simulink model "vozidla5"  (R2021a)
settings: Solver=VariableStepAuto  StartTime=0.0  StopTime=10.0  RelTol=1e-3
undefined symbols (not defined in the file or in its folder): ABK5, BC5, CC5, conds05, conds5, DC5
libraries: simulink x1

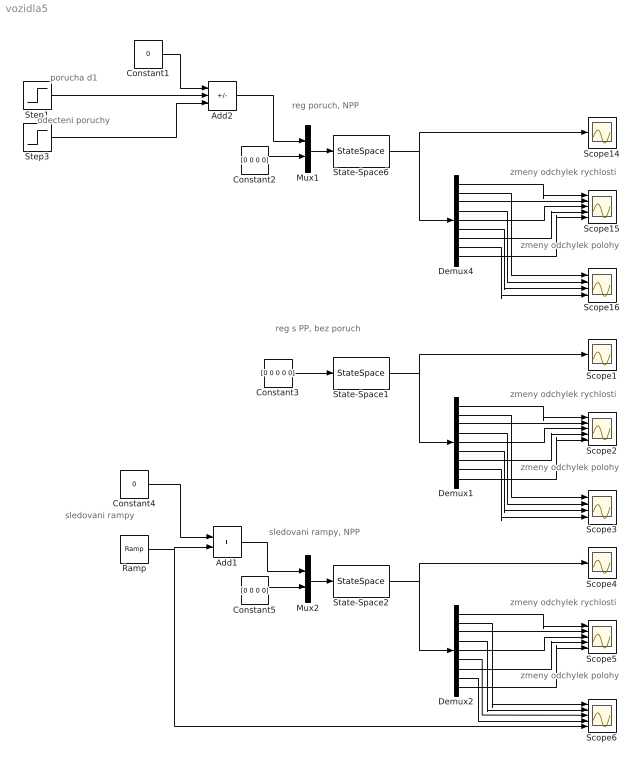
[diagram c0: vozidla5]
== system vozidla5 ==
  note: sledovani rampy
  note: reg poruch, NPP
  note: reg s PP, bez poruch
  note: odecteni poruchy
  note: porucha d1
  note: zmeny odchylek rychlosti
  note: zmeny odchylek polohy
  note: zmeny odchylek polohy
  note: zmeny odchylek rychlosti
  note: zmeny odchylek polohy
  note: sledovani rampy, NPP
  note: zmeny odchylek rychlosti
  Add1 : Sum
  Add2 : Sum  Inputs=++-
  Constant1 : Constant  Value=0
  Constant2 : Constant  Value=[0 0 0 0]
  Constant3 : Constant  Value=[0 0 0 0 0]
  Constant4 : Constant  Value=0
  Constant5 : Constant  Value=[0 0 0 0]
  Demux1 : Demux  Outputs=9
  Demux2 : Demux  Outputs=9
  Demux4 : Demux  Outputs=9
  Mux1 : Mux  Inputs=2
  Mux2 : Mux  Inputs=2
  Ramp : simulink/Sources/Ramp  slope=1  start=0  InitialOutput=0
  Scope1 : Scope
  Scope14 : Scope
  Scope{2,5..6,15} (4 alike) : Scope  NumInputPorts=5
  Scope16 : Scope  NumInputPorts=4
  Scope3 : Scope  NumInputPorts=4
  Scope4 : Scope
  State-Space1 : StateSpace  A=ABK5  B=BC5  C=CC5  D=DC5  InitialCondition=conds5
  State-Space2 : StateSpace  A=ABK5  B=BC5  C=CC5  D=DC5  InitialCondition=conds05
  State-Space6 : StateSpace  A=ABK5  B=BC5  C=CC5  D=DC5  InitialCondition=conds05
  Step1 : Step  Time=5  After=2  SampleTime=0
  Step3 : Step  Time=6  After=2  SampleTime=0
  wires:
  Demux4/5 -> Scope15/3
  Demux4/1 -> Scope15/1
  State-Space6/1 -> Demux4/1, Scope14/1
  Step1/1 -> Add2/2
  Add2/1 -> Mux1/1
  Mux1/1 -> State-Space6/1
  Step3/1 -> Add2/3
  Demux4/3 -> Scope15/2
  Constant1/1 -> Add2/1
  Constant2/1 -> Mux1/2
  Demux4/7 -> Scope15/4
  Demux4/9 -> Scope15/5
  Demux4/2 -> Scope16/1
  Demux4/4 -> Scope16/2
  Demux4/6 -> Scope16/3
  Demux4/8 -> Scope16/4
  Demux1/6 -> Scope3/3
  Demux1/4 -> Scope3/2
  Demux1/7 -> Scope2/4
  Demux1/8 -> Scope3/4
  Demux1/2 -> Scope3/1
  State-Space1/1 -> Demux1/1, Scope1/1
  Demux1/9 -> Scope2/5
  Demux1/3 -> Scope2/2
  Demux1/5 -> Scope2/3
  Demux1/1 -> Scope2/1
  Constant3/1 -> State-Space1/1
  Demux2/6 -> Scope6/3
  Demux2/4 -> Scope6/2
  Demux2/7 -> Scope5/4
  Demux2/8 -> Scope6/4
  Demux2/2 -> Scope6/1
  Constant5/1 -> Mux2/2
  Add1/1 -> Mux2/1
  State-Space2/1 -> Demux2/1, Scope4/1
  Demux2/3 -> Scope5/2
  Demux2/9 -> Scope5/5
  Demux2/5 -> Scope5/3
  Demux2/1 -> Scope5/1
  Constant4/1 -> Add1/1
  Mux2/1 -> State-Space2/1
  Ramp/1 -> Scope6/5, Add1/2
